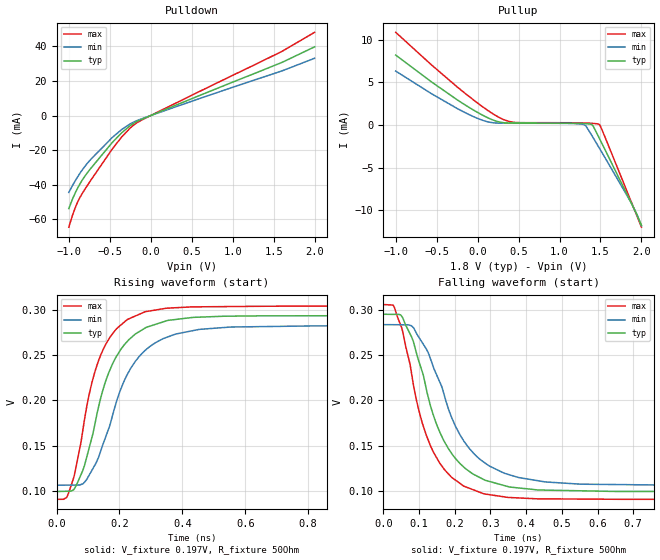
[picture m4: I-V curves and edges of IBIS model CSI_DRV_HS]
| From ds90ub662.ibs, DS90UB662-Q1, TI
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|   CSI_DRV_HS  Model
[Model]   CSI_DRV_HS
Model_type   Output
Polarity   Non-Inverting
Vmeas = 0.2
Vref = 0.2
Cref = 1pF
Rref = 50
|   typ   min   max
C_comp   0.533pF   0.500pF   0.567pF
[Voltage Range]   1.8   1.71   1.89
[Temperature Range]   27   105   -40
[Pullup Reference]   1.8   1.71   1.89
[Pulldown Reference]   0   0   0
[Power Clamp Reference]   1.8   1.71   1.89
[GND Clamp Reference]   0   0   0
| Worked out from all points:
|   slope of the pulldown table from 0 to 0.27 V, typ, clamps not added: 51.2 ohm
|   slope of the pullup table from 0 to 0.27 V, typ, clamps not added: 240 ohm
|   falling waveform, V_fixture 0.197V, R_fixture 50Ohm: 20-80 % time 106ps typ, 122ps min, 92.5ps max; typ from 0.295 V to 0.1 V
|   rising waveform, V_fixture 0.197V, R_fixture 50Ohm: 20-80 % time 107ps typ, 124ps min, 91.6ps max; typ from 0.1 V to 0.295 V
[Pulldown]
|   Voltage   I(typ)   I(min)   I(max)
-1V       -53.82mA   -44.47mA   -64.6mA
-955mV    -48.34mA   -40.49mA   -57.76mA
-913mV    -43.95mA   -37.09mA   -52.35mA
-877mV    -40.66mA   -34.36mA   -48.58mA
-826mV    -36.62mA   -30.81mA   -44.33mA
-736mV    -30.82mA   -25.57mA   -37.76mA
-454mV    -14.81mA   -12.05mA   -18.38mA
-349mV    -9.736mA   -7.898mA   -12.13mA
-214mV    -4.668mA   -3.904mA   -5.725mA
-40mV     -786.7uA   -671uA     -943.6uA
1.595V    30.62mA    25.72mA    36.98mA
2V        39.75mA    33.16mA    48.16mA
[Pullup]
|   Voltage   I(typ)   I(min)   I(max)
-1V       8.186mA    6.313mA    10.85mA
-562mV    5.036mA    3.655mA    7.03mA
-124mV    2.173mA    1.307mA    3.484mA
104mV     931uA      415.4uA    1.836mA
296mV     288.8uA    201.8uA    718.8uA
464mV     214.7uA    195.7uA    291.1uA
1.301V    155uA      41.19uA    234.5uA
1.397V    22.11uA    -1.28mA    184.5uA
1.481V    -1.468mA   -2.637mA   83.08uA
1.52V     -2.222mA   -3.27mA    -612.7uA
1.868V    -9.009mA   -9.009mA   -8.837mA
2V        -11.77mA   -11.83mA   -11.98mA
[Ramp]
R_load = 50
|   typ   min   max
dV/dt_r   0.117175/1.07008e-10   0.106147/1.24084e-10   0.12875/9.1735e-11
dV/dt_f   0.117128/1.06622e-10   0.10609/1.22337e-10   0.128737/9.23849e-11
[Falling Waveform]
V_fixture = 0.197V
V_fixture_min = 0.195V
V_fixture_max = 0.198V
R_fixture = 50Ohm
C_fixture = 0F
|   Time   V(typ)   V(min)   V(max)
0s        294.8mV    283.3mV    305.5mV
27.18ps   294.7mV    283.3mV    304.9mV
53.33ps   291.5mV    283.2mV    276.9mV
78.72ps   270mV      282.1mV    230mV
106.2ps   234.7mV    265.3mV    178.9mV
157.9ps   165mV      220.2mV    130.8mV
227.9ps   125.5mV    153.7mV    105.1mV
349.1ps   105mV      118.5mV    93.05mV
820.1ps   99.65mV    106.6mV    90.97mV
3.9ns     99.57mV    106.5mV    90.97mV
[Rising Waveform]
V_fixture = 0.197V
V_fixture_min = 0.195V
V_fixture_max = 0.198V
R_fixture = 50Ohm
C_fixture = 0F
|   Time   V(typ)   V(min)   V(max)
0s        99.57mV    106.5mV    90.97mV
33.12ps   99.85mV    106.6mV    93.6mV
65.82ps   108.6mV    106.7mV    133.1mV
110.8ps   156.8mV    121.9mV    217.1mV
157.9ps   222.9mV    161.3mV    262.7mV
201.8ps   254.7mV    210.1mV    282.2mV
236.4ps   268.8mV    235.6mV    290.7mV
349.1ps   287.5mV    269.3mV    301.4mV
820.1ps   293.1mV    282mV      303.7mV
3.9ns     294.9mV    283.4mV    305.5mV
